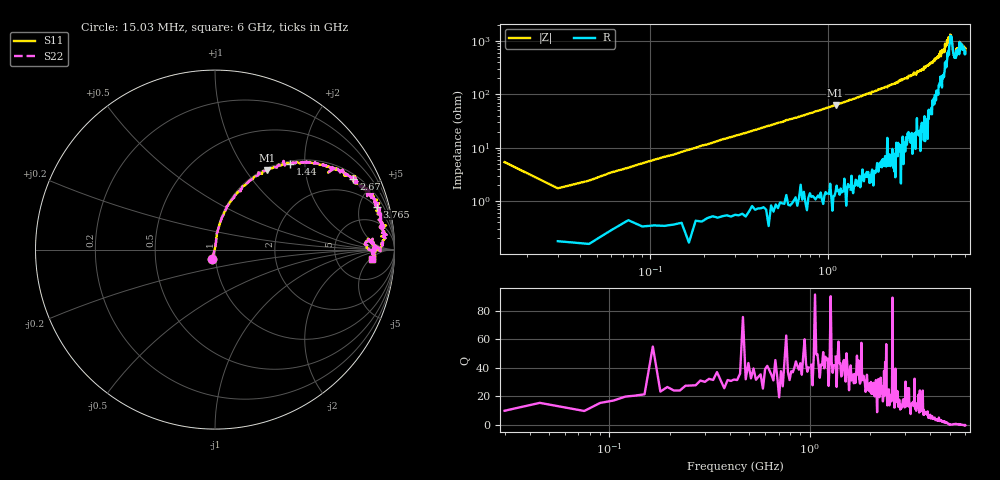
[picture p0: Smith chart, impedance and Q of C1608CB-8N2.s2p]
!	Network	Analyzer	HP8753E.07.74:	Oct	30	2002	Serial	No.	JP38451487
!	Hewlett-Packard
!	28	Aug	2009	7:47:49
!	Frequency	S11	S21	S12	S22
#	HZ	S	RI	R	50
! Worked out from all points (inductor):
!   400 points, 15.03 MHz to 6 GHz, reference 50 ohm
!   read as one part in series: L = 8.89 nH near 45.03 MHz
!   highest Q = 48.1 at 1.11 GHz (marker M1), where L = 9.01 nH
!   self-resonance near 5.018 GHz
!   S11 on the Smith chart (normalised r, x): 15.03 MHz: 0.97, -0.10; 1.44 GHz: 1.05, +1.69; 2.67 GHz: 1.21, +3.80; 3.765 GHz: 1.94, +7.16; 6 GHz: 13, -6
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1.502992e7  -0.0151 -0.0517  1.02 0.0517  1.02 0.0517  -0.0151 -0.0517
3.002985e7  0.00213 0.0172  0.998 -0.0172  0.998 -0.0172  0.00213 0.0172
1.050295e8  0.00689 0.0586  0.993 -0.0586  0.993 -0.0586  0.00689 0.0586
2.550287e8  0.025 0.139  0.975 -0.139  0.975 -0.139  0.025 0.139
5.850271e8  0.107 0.29  0.893 -0.29  0.893 -0.29  0.107 0.29
1.020025e9  0.253 0.423  0.747 -0.423  0.747 -0.423  0.253 0.423
1.110024e9  0.288 0.441  0.712 -0.441  0.712 -0.441  0.288 0.441
1.440023e9  0.42 0.479  0.58 -0.479  0.58 -0.479  0.42 0.479
2.01002e9  0.616 0.465  0.384 -0.465  0.384 -0.465  0.616 0.465
2.670017e9  0.771 0.393  0.229 -0.393  0.229 -0.393  0.771 0.393
3.015015e9  0.835 0.355  0.165 -0.355  0.165 -0.355  0.835 0.355
3.765011e9  0.902 0.239  0.098 -0.239  0.098 -0.239  0.902 0.239
4.00501e9  0.928 0.196  0.0718 -0.196  0.0718 -0.196  0.928 0.196
4.935005e9  0.932 0.0209  0.0675 -0.0209  0.0675 -0.0209  0.932 0.0209
5.010005e9  0.919 0.00891  0.0812 -0.00891  0.0812 -0.00891  0.919 0.00891
5.205004e9  0.834 0.0294  0.166 -0.0294  0.166 -0.0294  0.834 0.0294
5.355003e9  0.884 0.0394  0.116 -0.0394  0.116 -0.0394  0.884 0.0394
5.535002e9  0.864 0.045  0.136 -0.045  0.136 -0.045  0.864 0.045
5.565002e9  0.907 0.0119  0.0935 -0.0119  0.0935 -0.0119  0.907 0.0119
5.595002e9  0.875 0.0316  0.125 -0.0316  0.125 -0.0316  0.875 0.0316
5.685002e9  0.899 0.00333  0.101 -0.00333  0.101 -0.00333  0.899 0.00333
6e9  0.875 -0.0511  0.125 0.0511  0.125 0.0511  0.875 -0.0511
